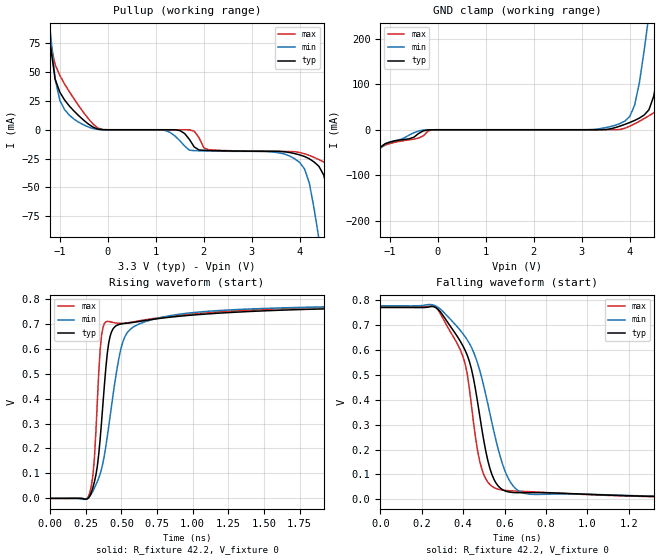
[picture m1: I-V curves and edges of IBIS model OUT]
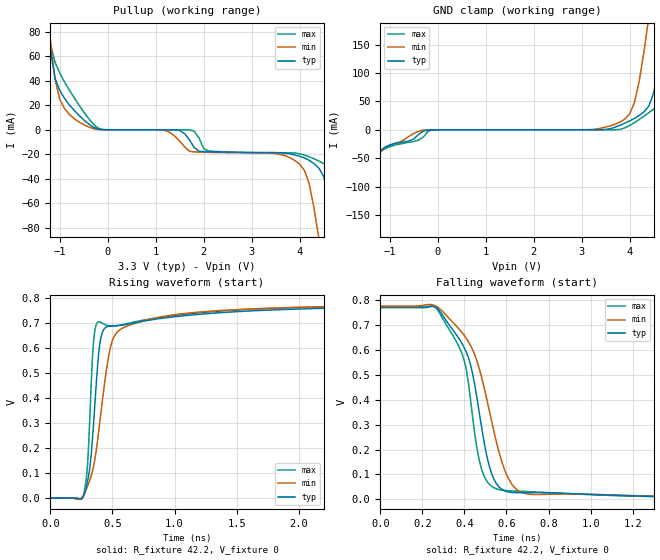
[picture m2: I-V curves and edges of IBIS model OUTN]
|   IBIS File of SG2016HGN C
|   HCSL Zdiff=85, Vcc=3.3V, fo<=212.5MHz
[IBIS Ver]   3.2
[File Name]   sg2016hgn_85_33v.ibs
[File Rev]   1.0
[Date]   Jan. 27, 2023
[Source]
[Notes]
Created by Minoru Kozaki
[Disclaimer]
Seiko Epson Corporation makes no warranty with respect to the
information contained herein.
[Copyright]
Copyright(C) 2023, Seiko Epson Corporation. All rights reserved.
|   Component
[Component]   SG2016HGN
[Manufacturer]  Seiko Epson Corporation
[Package]
R_pkg   8.9m   NA   NA
L_pkg   197p   NA   NA
C_pkg   267f   NA   NA
[Pin]   signal_name   model_name   R_pin   L_pin   C_pin
1   OE/ST   NC
2   NC   NC
3   GND   GND
4   OUT   OUT   8.9m   197p   267f
5   OUTN   OUTN   9.9m   222p   245f
6   VCC   POWER
[Diff Pin] inv_pin  vdiff  tdelay_typ
4   5   0   0
| Models and submodels in the file (2): OUT (Open_source), OUTN (Open_source)
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|   Model OUT
[Model]   OUT
Model_type   Open_source
Polarity   Non-Inverting
Vref = 0
Vmeas = 0.4
Rref = 42.2
Cref = 0
C_comp   12.0p   12.0p   12.0p
[Temperature Range]   25   105   -40
[Voltage Range]   3.3   2.97   3.63
[Pullup Reference]   3.3   2.97   3.63
[GND Clamp Reference]   0   0   0
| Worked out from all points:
|   GND clamp passes 1 mA (typ) near -0.23 V on its own axis
|   falling waveform, R_fixture 42.2, V_fixture 0: 20-80 % time 121ps typ, 152ps min, 105ps max; typ from 0.771 V to 0 V
|   rising waveform, R_fixture 42.2, V_fixture 0: 20-80 % time 73.2ps typ, 133ps min, 45.5ps max; typ from 0 V to 0.77 V
[Pullup]
-3.3V     2.129A     2.051A     2.213A
-1.3V     133.8mA    151.4mA    127.3mA
-1.2V     73.93mA    85.63mA    76.3mA
-1.1V     43.93mA    44mA       56.48mA
-1V       32.41mA    25.29mA    47.02mA
-200mV    439.2uA    190.2uA    1.262mA
3.8V      -19.8mA    -22.97mA   -18.85mA
4.1V      -23.15mA   -33.96mA   -20.77mA
4.4V      -31.71mA   -94.59mA   -25.88mA
4.8V      -112.9mA   -198.6mA   -39.07mA
5.1V      -198.1mA   -276.7mA   -106.3mA
6.6V      -624.9mA   -668.6mA   -567.9mA
[GND Clamp]
-3.3V     -623.5mA   -581mA     -670mA
-1.9V     -225.2mA   -215.9mA   -236.7mA
-1.2V     -38.35mA   -41.07mA   -39.76mA
-200mV    -326.8uA   -114.9uA   -2.508mA
3.9V      11.86mA    19.19mA    3.412mA
4.1V      20.39mA    53.69mA    12.92mA
4.4V      43.93mA    253.5mA    30.83mA
4.5V      73.93mA    333.2mA    37.35mA
4.7V      214.5mA    494.1mA    53.26mA
4.8V      299.8mA    575.1mA    67.95mA
5.1V      561.2mA    820.3mA    269.9mA
6.6V      2.129A     2.437A     1.773A
[Falling Waveform]
R_fixture = 42.2
V_fixture = 0
V_fixture_min = 0
V_fixture_max = 0
0s        770.9mV    777.7mV    775.4mV
260ps     773.8mV    779.9mV    776mV
370ps     656.9mV    695mV      628.2mV
420ps     578.7mV    640.6mV    502.7mV
490ps     283.8mV    487.5mV    122.1mV
530ps     122mV      342.2mV    58.87mV
570ps     52.99mV    199.1mV    40.77mV
640ps     27.75mV    55.1mV     34.08mV
730ps     27.13mV    20.42mV    30.68mV
4ns       261uV      394uV      211uV
[Rising Waveform]
R_fixture = 42.2
V_fixture = 0
V_fixture_min = 0
V_fixture_max = 0
0s        96uV       137uV      91uV
280ps     11.68mV    11.17mV    27.75mV
310ps     66.55mV    41.94mV    163.4mV
350ps     236.5mV    97.51mV    594.8mV
370ps     380.4mV    143.1mV    684.9mV
390ps     521.7mV    208.1mV    707.3mV
430ps     667.1mV    370.5mV    706.1mV
510ps     699.9mV    627.6mV    701.4mV
720ps     717.2mV    716.7mV    720.1mV
4ns       770.1mV    776.7mV    774.8mV
[Ramp]
R_load = 42.2
dV/dt_r   0.46957/74.94p   0.47278/136.74p   0.47293/46.11p
dV/dt_f   0.46957/126.32p   0.47278/156.69p   0.47293/110.44p
|   Model OUTN
[Model]   OUTN
Model_type   Open_source
Polarity   Inverting
Vref = 0
Vmeas = 0.4
Rref = 42.2
Cref = 0
C_comp   12.0p   12.0p   12.0p
[Temperature Range]   25   105   -40
[Voltage Range]   3.3   2.97   3.63
[Pullup Reference]   3.3   2.97   3.63
[GND Clamp Reference]   0   0   0
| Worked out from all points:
|   GND clamp passes 1 mA (typ) near -0.23 V on its own axis
|   falling waveform, R_fixture 42.2, V_fixture 0: 20-80 % time 117ps typ, 149ps min, 100ps max; typ from 0.77 V to 0 V
|   rising waveform, R_fixture 42.2, V_fixture 0: 20-80 % time 73.1ps typ, 135ps min, 45ps max; typ from 0 V to 0.769 V
[Pullup]
-3.3V     1.492A     1.466A     1.533A
-1.3V     109.2mA    122.6mA    105.6mA
-1.2V     65.38mA    73.61mA    70.08mA
-1.1V     42mA       40.79mA    54.93mA
-1V       31.82mA    24.61mA    46.12mA
-200mV    438uA      190uA      1.253mA
3.8V      -19.74mA   -22.88mA   -18.84mA
4.1V      -23.01mA   -33.36mA   -20.66mA
4.4V      -31.32mA   -89.1mA    -25.6mA
4.8V      -105.6mA   -187.2mA   -38.24mA
5.1V      -185.6mA   -260.8mA   -98.76mA
6.6V      -586mA     -630.5mA   -529.2mA
[GND Clamp]
-3.3V     -584.5mA   -547.9mA   -624.3mA
-1.8V     -184.4mA   -179.1mA   -191.7mA
-1.2V     -37.27mA   -39.78mA   -38.69mA
-200mV    -326uA     -114.8uA   -2.462mA
3.8V      8.017mA    13.68mA    676.8uA
4.1V      20.13mA    48.7mA     12.72mA
4.4V      42mA       200.5mA    30.28mA
4.5V      65.38mA    262.7mA    36.66mA
4.7V      167.7mA    388.1mA    52.04mA
4.8V      232.7mA    451.2mA    64.06mA
5.1V      432.3mA    641.4mA    207mA
6.6V      1.492A     1.742A     1.284A
[Falling Waveform]
R_fixture = 42.2
V_fixture = 0
V_fixture_min = 0
V_fixture_max = 0
0s        769.6mV    776.3mV    773.9mV
260ps     772.4mV    778mV      773.3mV
370ps     651mV      688.2mV    620.7mV
430ps     537.5mV    616.9mV    393.9mV
480ps     298mV      495.9mV    126mV
520ps     128.2mV    349.5mV    59.14mV
560ps     54.22mV    203.8mV    40.4mV
630ps     27.35mV    55.77mV    33.82mV
720ps     26.89mV    20.01mV    30.6mV
4ns       256uV      385uV      208uV
[Rising Waveform]
R_fixture = 42.2
V_fixture = 0
V_fixture_min = 0
V_fixture_max = 0
0s        88uV       139uV      90uV
270ps     9.587mV    13.85mV    17.44mV
300ps     67.13mV    48.24mV    135.7mV
330ps     178.7mV    90.1mV     465.2mV
350ps     311.2mV    131.4mV    638.2mV
390ps     582.6mV    268.5mV    705.8mV
430ps     675mV      433.4mV    697.1mV
500ps     689.8mV    631.3mV    688.5mV
740ps     707.5mV    708.5mV    711.5mV
4ns       768.7mV    775.1mV    773.3mV
[Ramp]
R_load = 42.2
dV/dt_r   0.46946/75.16p   0.47268/140.02p   0.47277/45.83p
dV/dt_f   0.46946/122.93p   0.47268/154.24p   0.47277/106.56p
